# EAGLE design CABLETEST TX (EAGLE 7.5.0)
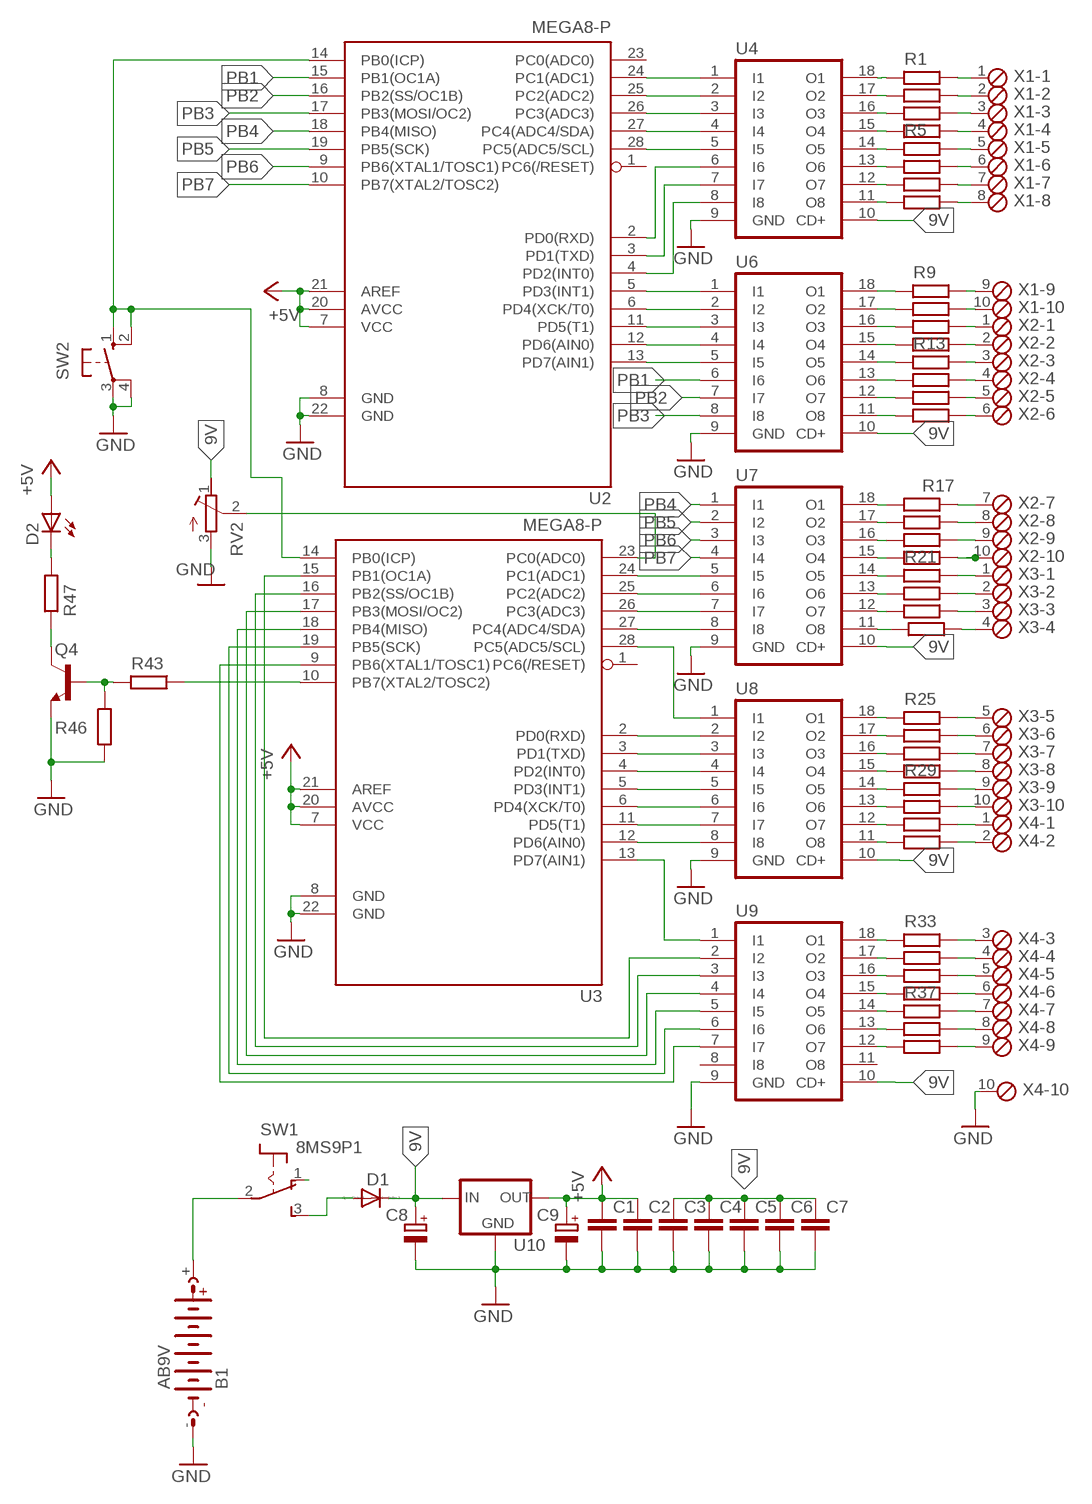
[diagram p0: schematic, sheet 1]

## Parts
B1  AB9V  [AB9V]
C1  C-EUC1206  [C1206]
C2  C-EUC1206  [C1206]
C3  C-EUC1206  [C1206]
C4  C-EUC1206  [C1206]
C5  C-EUC1206  [C1206]
C6  C-EUC1206  [C1206]
C7  C-EUC1206  [C1206]
C8  CPOL-EUE2-5  [E2-5]
C9  CPOL-EUE2-5  [E2-5]
D1  1N4004  [DO41-10]
D2  LED5MM  [LED5MM]
Q4  BC337  [TO92]
R1  R-EU_R1206  [R1206]
R2  R-EU_R1206  [R1206]
R3  R-EU_R1206  [R1206]
R4  R-EU_R1206  [R1206]
R5  R-EU_R1206  [R1206]
R6  R-EU_R1206  [R1206]
R7  R-EU_R1206  [R1206]
R8  R-EU_R1206  [R1206]
R9  R-EU_R1206  [R1206]
R10  R-EU_R1206  [R1206]
R11  R-EU_R1206  [R1206]
R12  R-EU_R1206  [R1206]
R13  R-EU_R1206  [R1206]
R14  R-EU_R1206  [R1206]
R15  R-EU_R1206  [R1206]
R16  R-EU_R1206  [R1206]
R17  R-EU_R1206  [R1206]
R18  R-EU_R1206  [R1206]
R19  R-EU_R1206  [R1206]
R20  R-EU_R1206  [R1206]
R21  R-EU_R1206  [R1206]
R22  R-EU_R1206  [R1206]
R23  R-EU_R1206  [R1206]
R24  R-EU_R1206  [R1206]
R25  R-EU_R1206  [R1206]
R26  R-EU_R1206  [R1206]
R27  R-EU_R1206  [R1206]
R28  R-EU_R1206  [R1206]
R29  R-EU_R1206  [R1206]
R30  R-EU_R1206  [R1206]
R31  R-EU_R1206  [R1206]
R32  R-EU_R1206  [R1206]
R33  R-EU_R1206  [R1206]
R34  R-EU_R1206  [R1206]
R35  R-EU_R1206  [R1206]
R36  R-EU_R1206  [R1206]
R37  R-EU_R1206  [R1206]
R38  R-EU_R1206  [R1206]
R39  R-EU_R1206  [R1206]
R43  R-EU_R1206  [R1206]
R46  R-EU_R1206  [R1206]
R47  R-EU_R1206  [R1206]
RV2  R-TRIMM-3386-F  [R-TRIMM-3386F]
SW1  8MS9P1  [8MS9]
SW2  10-XX  [B3F-10XX]
U2  MEGA8-P  [DIL28-3]
U3  MEGA8-P  [DIL28-3]
U4  ULN2803A  [DIL18]
U6  ULN2803A  [DIL18]
U7  ULN2803A  [DIL18]
U8  ULN2803A  [DIL18]
U9  ULN2803A  [DIL18]
U10  78XXL  [78XXL]
X1  MPT10  [10POL254]
X2  MPT10  [10POL254]
X3  MPT10  [10POL254]
X4  MPT10  [10POL254]

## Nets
9V: C3.1 C4.1 C5.1 C6.1 C7.1 C8.+ D1.C RV2.1(A) U4.10(CD+) U6.10(CD+) U7.10(CD+) U8.10(CD+) U9.10(CD+) U10.IN
+5V: C1.1 C2.1 C9.+ D2.A U2.7(VCC) U2.20(AVCC) U2.21(AREF) U3.7(VCC) U3.20(AVCC) U3.21(AREF) U10.OUT
GND: B1.- C1.2 C2.2 C3.2 C4.2 C5.2 C6.2 C7.2 C8.- C9.- Q4.1(E) R46.2 RV2.3(E) SW2.3(P) SW2.4(P1) U2.8(GND) U2.22(GND) U3.8(GND) U3.22(GND) U4.9(GND) U6.9(GND) U7.9(GND) U8.9(GND) U9.9(GND) U10.GND X4.10
N$1: U2.24(PC1(ADC1)) U4.1(I1)
N$2: U2.25(PC2(ADC2)) U4.2(I2)
N$3: U2.26(PC3(ADC3)) U4.3(I3)
N$4: U2.27(PC4(ADC4/SDA)) U4.4(I4)
N$5: U2.28(PC5(ADC5/SCL)) U4.5(I5)
N$6: U2.2(PD0(RXD)) U4.6(I6)
N$7: U2.3(PD1(TXD)) U4.7(I7)
N$8: U2.4(PD2(INT0)) U4.8(I8)
N$9: U2.5(PD3(INT1)) U6.1(I1)
N$10: U2.6(PD4(XCK/T0)) U6.2(I2)
N$11: U2.11(PD5(T1)) U6.3(I3)
N$12: U2.12(PD6(AIN0)) U6.4(I4)
N$13: U2.13(PD7(AIN1)) U6.5(I5)
N$14: U3.24(PC1(ADC1)) U7.5(I5)
N$15: U3.25(PC2(ADC2)) U7.6(I6)
N$16: U3.26(PC3(ADC3)) U7.7(I7)
N$17: U3.27(PC4(ADC4/SDA)) U7.8(I8)
N$18: U3.28(PC5(ADC5/SCL)) U8.1(I1)
N$19: U3.2(PD0(RXD)) U8.2(I2)
N$20: U3.3(PD1(TXD)) U8.3(I3)
N$21: U3.4(PD2(INT0)) U8.4(I4)
N$22: U3.5(PD3(INT1)) U8.5(I5)
N$23: U3.6(PD4(XCK/T0)) U8.6(I6)
N$24: U3.11(PD5(T1)) U8.7(I7)
N$25: U3.12(PD6(AIN0)) U8.8(I8)
N$26: U3.13(PD7(AIN1)) U9.1(I1)
N$27: U3.15(PB1(OC1A)) U9.2(I2)
N$28: U3.16(PB2(SS/OC1B)) U9.3(I3)
N$29: U3.17(PB3(MOSI/OC2)) U9.4(I4)
N$30: U3.18(PB4(MISO)) U9.5(I5)
N$31: U3.19(PB5(SCK)) U9.6(I6)
N$32: U3.9(PB6(XTAL1/TOSC1)) U9.7(I7)
N$33: Q4.3(C) R47.2
N$34: D1.A SW1.3(S)
N$35: RV2.2(S) U3.23(PC0(ADC0))
N$36: D2.K(C) R47.1
N$38: Q4.2(B) R43.2 R46.1
N$39: R43.1 U3.10(PB7(XTAL2/TOSC2))
N$40: SW2.1(S) SW2.2(S1) U2.14(PB0(ICP)) U3.14(PB0(ICP))
N$41: R1.2 U4.18(O1)
N$42: R1.1 X1.1
N$43: R2.2 U4.17(O2)
N$44: R2.1 X1.2
N$45: R3.2 U4.16(O3)
N$46: R3.1 X1.3
N$47: R4.1 X1.4
N$48: R5.1 X1.5
N$49: R6.1 X1.6
N$50: R8.2 U4.11(O8)
N$51: R4.2 U4.15(O4)
N$52: R5.2 U4.14(O5)
N$53: R6.2 U4.13(O6)
N$54: R7.2 U4.12(O7)
N$55: R7.1 X1.7
N$56: R8.1 X1.8
N$57: R9.1 X1.9
N$58: R10.1 X1.10
N$59: R11.1 X2.1
N$60: R12.1 X2.2
N$61: R13.1 X2.3
N$62: R14.1 X2.4
N$63: R15.1 X2.5
N$64: R16.1 X2.6
N$65: R17.2 U7.18(O1)
N$66: R18.2 U7.17(O2)
N$67: R19.2 U7.16(O3)
N$68: R20.2 U7.15(O4)
N$69: R21.2 U7.14(O5)
N$70: R22.2 U7.13(O6)
N$71: R23.2 U7.12(O7)
N$72: R24.2 U7.11(O8)
N$73: R9.2 U6.18(O1)
N$74: R10.2 U6.17(O2)
N$75: R11.2 U6.16(O3)
N$76: R12.2 U6.15(O4)
N$77: R13.2 U6.14(O5)
N$78: R14.2 U6.13(O6)
N$79: R15.2 U6.12(O7)
N$80: R16.2 U6.11(O8)
N$81: R25.1 X3.5
N$82: R17.1 X2.7
N$83: R26.1 X3.6
N$84: R18.1 X2.8
N$85: R27.1 X3.7
N$86: R19.1 X2.9
N$87: R20.1 X2.10
N$88: R21.1 X3.1
N$89: R22.1 X3.2
N$90: R28.1 X3.8
N$91: R29.1 X3.9
N$92: R30.1 X3.10
N$93: R31.1 X4.1
N$94: R32.1 X4.2
N$95: R23.1 X3.3
N$96: R24.1 X3.4
N$97: SW1.1(O)
N$98: R25.2 U8.18(O1)
N$99: R33.1 X4.3
N$100: R26.2 U8.17(O2)
N$101: R34.1 X4.4
N$102: R27.2 U8.16(O3)
N$103: R35.1 X4.5
N$104: R36.1 X4.6
N$105: R37.1 X4.7
N$106: R38.1 X4.8
N$107: R28.2 U8.15(O4)
N$108: R29.2 U8.14(O5)
N$109: R30.2 U8.13(O6)
N$110: R31.2 U8.12(O7)
N$111: R32.2 U8.11(O8)
N$112: R39.1 X4.9
N$113: B1.+ SW1.2(P)
N$114: R33.2 U9.18(O1)
N$123: R34.2 U9.17(O2)
N$124: R35.2 U9.16(O3)
N$125: R36.2 U9.15(O4)
N$126: R37.2 U9.14(O5)
N$127: R38.2 U9.13(O6)
N$128: R39.2 U9.12(O7)
PB1: U2.15(PB1(OC1A)) U6.6(I6)
PB2: U2.16(PB2(SS/OC1B)) U6.7(I7)
PB3: U2.17(PB3(MOSI/OC2)) U6.8(I8)
PB4: U2.18(PB4(MISO)) U7.1(I1)
PB5: U2.19(PB5(SCK)) U7.2(I2)
PB6: U2.9(PB6(XTAL1/TOSC1)) U7.3(I3)
PB7: U2.10(PB7(XTAL2/TOSC2)) U7.4(I4)
Unconnected: U2.1(PC6(/RESET)) U2.23(PC0(ADC0)) U3.1(PC6(/RESET)) U9.8(I8) U9.11(O8)

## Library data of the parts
B1 = battery:AB9V: 9-V BATTERY CLIP
C1-C7 = rcl:C-EU: CAPACITOR, European symbol
C8 C9 = rcl:CPOL-EU: POLARIZED CAPACITOR, European symbol
D1 = diode:1N4004: DIODE
D2 = led:LED: LED
Q4 = transistor:BC337: NPN TRANSISTOR
R1-R39 R43 R46 R47 = rcl:R-EU_: RESISTOR, European symbol
RV2 = rcl:R-TRIMM-3386-F
SW1 = switch:8MS9P1
SW2 = switch-omron:10-XX: OMRON SWITCH; MPN: B3F-1000; OC_FARNELL: 176432; OC_NEWARK: 36M3542
U2 U3 = atmel:MEGA8-P: MICROCONTROLLER 8 Kbytes FLASH, 1 kbytes SRAM, 512 bytes EEPROM, USART, 4-channel 10 bit ADC, 2-channel 8 bit ADC Pin compatible with Atmega48, ATMega88, ATMega168 Source: avr.lbr; OC_FARNELL: unknown; OC_NEWARK: unknown
U4 U6-U9 = uln-udn:ULN2803A: DRIVER ARRAY
U10 = v-reg:78XXL: VOLTAGE REGULATOR
X1-X4 = con-phoenix-254:MPT10: PHOENIX CONNECTOR; OC_FARNELL: unknown; OC_NEWARK: unknown

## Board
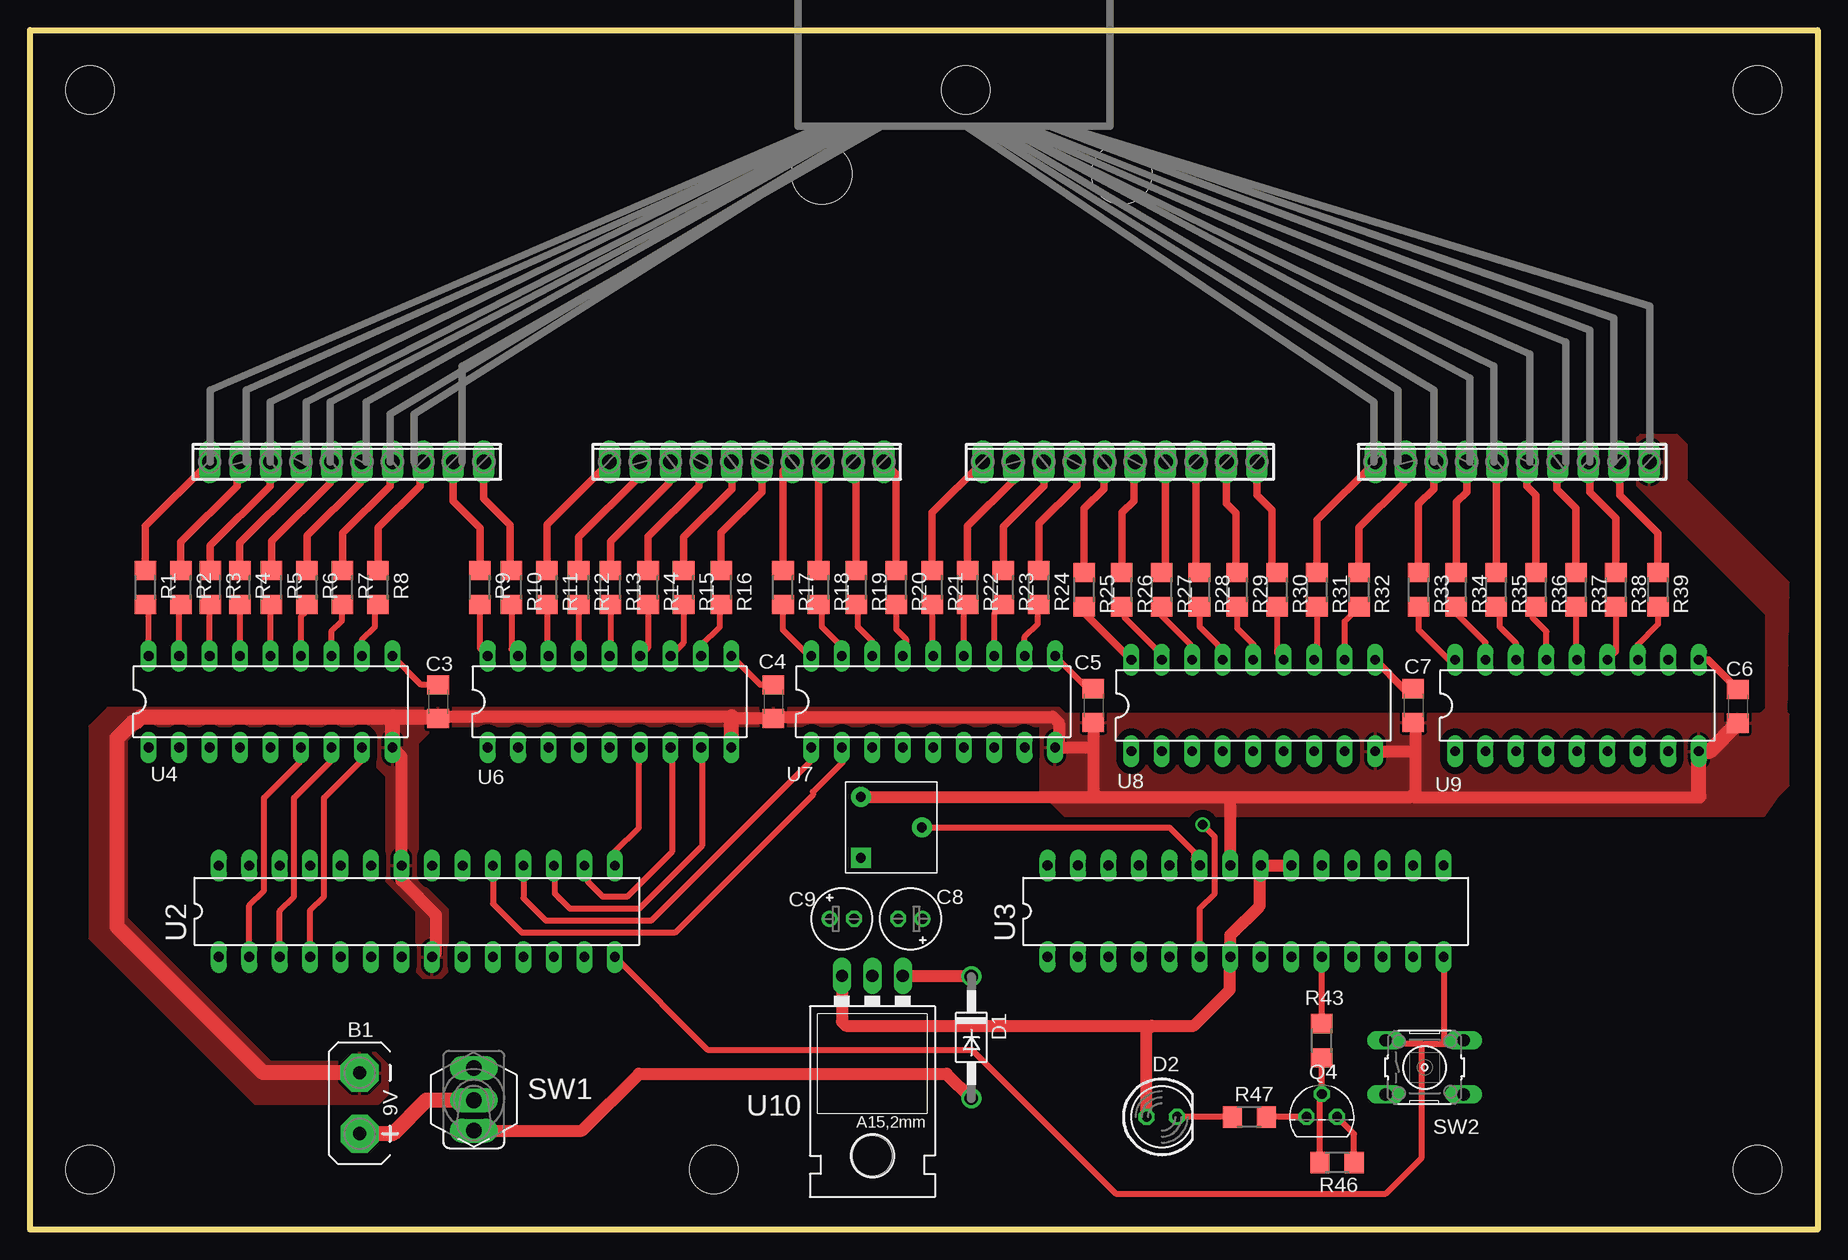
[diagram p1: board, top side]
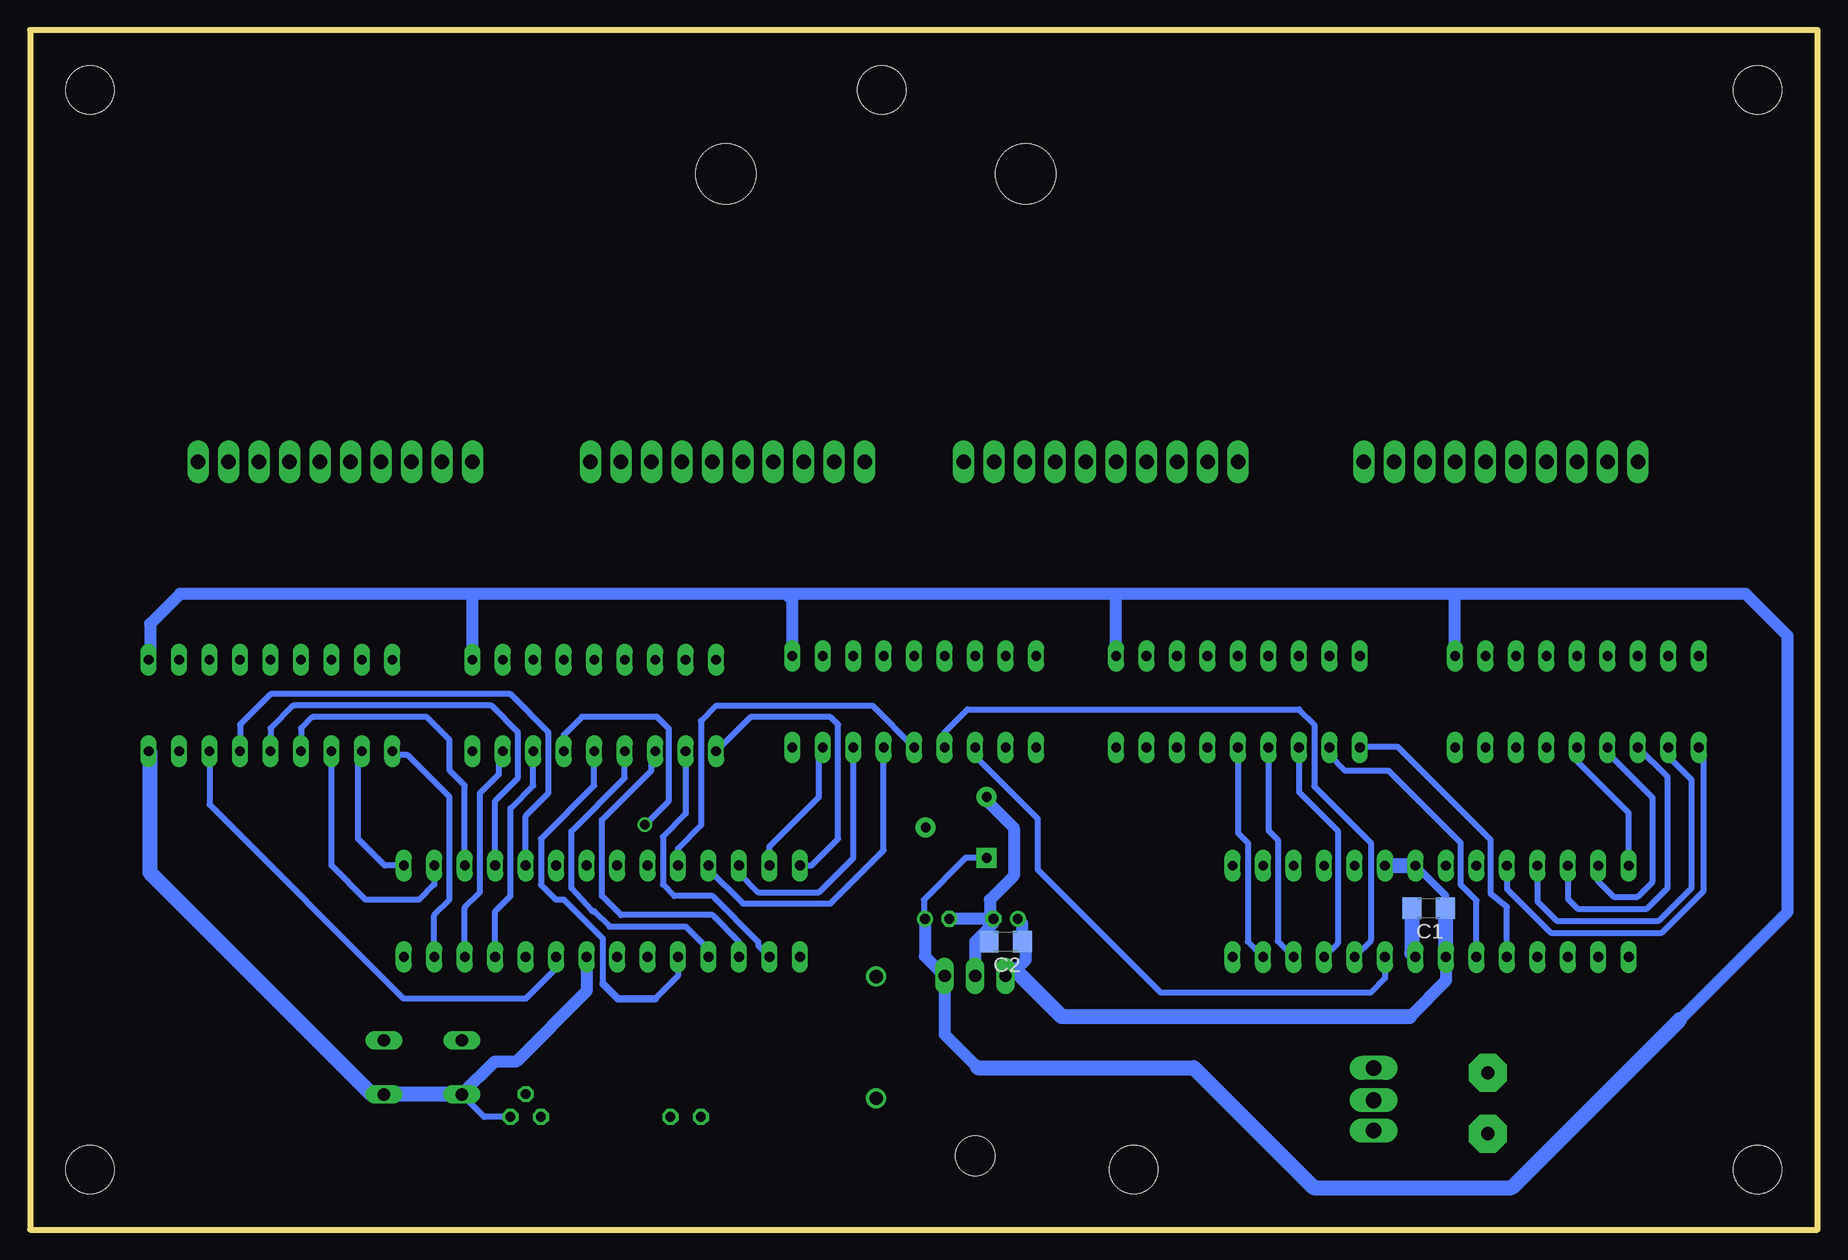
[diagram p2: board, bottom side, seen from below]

Size 149 x 100 mm. Coordinates in mm from the lower left corner, seen from the top.
Outline: 0,0 0,100 149,100 149,0 0,0
Copper layers (1*16): Top 0.035mm / dielectric 1.5mm / Bottom 0.035mm
Design rules "default": minimum track width 10mil, minimum drill 24mil, track to track 8mil, track to pad 8mil, pad to pad 8mil, via to via 8mil, smd to smd 8mil, copper to edge 40mil, drill to drill 8mil, minimum pad ring 10mil, minimum via ring 8mil, stop-mask expansion 4mil, vias tented up to drill 0mil, thermal gap 10mil
Holes 4 mm at 5,5 57,5 144,5 5,95 78,95 144,95
Holes 5 mm at 66,88 91,88

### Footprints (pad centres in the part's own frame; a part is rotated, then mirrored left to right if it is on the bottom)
AB9V = drill 1.118 pad 3.15 octagon: + 0,2.54; - 0,-2.54
C1206 = smd 1.6 x 1.8: 1 -1.4,0; 2 1.4,0
E2-5 = drill 0.813 pad 1.27: + -1.016,0 | drill 0.813 pad 1.27 octagon: - 1.016,0
DO41-10 = drill 1.118: A 5.08,0; C -5.08,0
LED5MM = drill 0.813 octagon: A -1.27,0; K 1.27,0
TO92 = drill 0.813 octagon: 1 1.27,0; 2 0,1.905; 3 -1.27,0
R1206 = smd 1.6 x 1.803: 1 -1.422,0; 2 1.422,0
R-TRIMM-3386F = drill 0.8 pad 1.676 square: 1 0,0 | drill 0.8 pad 1.676: 2 5.08,2.54; 3 0,5.08
8MS9 = drill 1.295 pad 2 long: 1 -3,5.346 | drill 1.3 pad 2 long: 2 -3,2.654; 3 -3,0.114
B3F-10XX = drill 1.016 long: 1 -3.251,2.261; 2 3.251,2.261; 3 -3.251,-2.261; 4 3.251,-2.261
DIL28-3 = drill 0.813 long: 1 -16.51,-3.81; 2 -13.97,-3.81; 3 -11.43,-3.81; 4 -8.89,-3.81; 5 -6.35,-3.81; 6 -3.81,-3.81; 7 -1.27,-3.81; 8 1.27,-3.81; 9 3.81,-3.81; 10 6.35,-3.81; 11 8.89,-3.81; 12 11.43,-3.81; 13 13.97,-3.81; 14 16.51,-3.81; 15 16.51,3.81; 16 13.97,3.81; 17 11.43,3.81; 18 8.89,3.81; 19 6.35,3.81; 20 3.81,3.81; 21 1.27,3.81; 22 -1.27,3.81; 23 -3.81,3.81; 24 -6.35,3.81; 25 -8.89,3.81; 26 -11.43,3.81; 27 -13.97,3.81; 28 -16.51,3.81
DIL18 = drill 0.813 long: 1 -10.16,-3.81; 2 -7.62,-3.81; 3 -5.08,-3.81; 4 -2.54,-3.81; 5 0,-3.81; 6 2.54,-3.81; 7 5.08,-3.81; 8 7.62,-3.81; 9 10.16,-3.81; 10 10.16,3.81; 11 7.62,3.81; 12 5.08,3.81; 13 2.54,3.81; 14 0,3.81; 15 -2.54,3.81; 16 -5.08,3.81; 17 -7.62,3.81; 18 -10.16,3.81
78XXL = drill 1.016 long: GND 0,-3.81; IN -2.54,-3.81; OUT 2.54,-3.81 | hole 3.302: 0,11.176
10POL254 = drill 1.2 long: 1 -11.43,0; 2 -8.89,0; 3 -6.35,0; 4 -3.81,0; 5 -1.27,0; 6 1.27,0; 7 3.81,0; 8 6.35,0; 9 8.89,0; 10 11.43,0

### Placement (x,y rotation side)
B1  27.48,10.53 180 top
C1  32.42,26.79 180 bottom
C2  67.67,24 180 bottom
C3  34.02,44 270 top
C4  61.96,44 270 top
C5  88.63,43.68 270 top
C6  142.35,43.61 270 top
C7  115.3,43.68 270 top
C8  73.39,25.9 180 top
C9  67.67,25.9 0 top
D1  78.47,16.02 270 top
D2  94.34,9.39 0 top
Q4  107.68,9.39 0 top
R1  9.61,53.52 270 top
R2  12.57,53.52 270 top
R3  15.03,53.52 270 top
R4  17.49,53.52 270 top
R5  20.13,53.52 270 top
R6  23.09,53.52 270 top
R7  26.05,53.52 270 top
R8  29.01,53.52 270 top
R9  37.49,53.52 270 top
R10  40.13,53.52 270 top
R11  43.09,53.52 270 top
R12  45.73,53.52 270 top
R13  48.38,53.52 270 top
R14  51.52,53.52 270 top
R15  54.48,53.52 270 top
R16  57.62,53.52 270 top
R17  62.77,53.52 270 top
R18  65.73,53.52 270 top
R19  68.87,53.52 270 top
R20  72.2,53.52 270 top
R21  75.2,53.52 270 top
R22  78.17,53.52 270 top
R23  81.12,53.52 270 top
R24  84.08,53.52 270 top
R25  87.87,53.34 270 top
R26  91.01,53.34 270 top
R27  94.34,53.34 270 top
R28  97.48,53.34 270 top
R29  100.62,53.34 270 top
R30  103.95,53.34 270 top
R31  107.27,53.34 270 top
R32  110.78,53.34 270 top
R33  115.75,53.34 270 top
R34  118.89,53.34 270 top
R35  122.22,53.34 270 top
R36  125.54,53.34 270 top
R37  128.87,53.34 270 top
R38  132.19,53.34 270 top
R39  135.7,53.34 270 top
R43  107.68,15.74 270 top
R46  108.95,5.58 0 top
R47  101.65,9.39 0 top
RV2  69.26,30.98 0 top
SW1  40,8.12 0 top
SW2  116.25,13.52 0 top
U2  32.24,26.53 0 top
U3  101.33,26.54 0 top
U4  20.05,44 0 top
U6  48.31,44 0 top
U7  75.3,44 0 top
U8  101.97,43.68 0 top
U9  128.95,43.68 0 top
U10  70.22,17.33 180 top
X1  26.4,64 0 top
X2  59.74,64 0 top
X3  90.85,64 0 top
X4  123.56,64 0 top

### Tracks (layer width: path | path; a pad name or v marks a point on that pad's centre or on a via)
9V
  Top 0.5: C3.1 32.62,45.4 U4.10 | C4.1 60.88,45.4 U6.10 | C5.1 88.18,45.08 U7.10
  Top 0.61: C7.1 114.53,45.08 U8.10 | U9.10 139.88,47.49 C6.1
  Top 1.016: U10.IN 78.43,21.14 D1.C
  Bottom 0.5: RV2.1 71.02,30.98 74.5,27.5 74.5,25.99 C8.+
  Bottom 1.016: 70,13.5 72.75,16.25 U10.IN 74.41,22.79 C8.+ | 11.5,17.5 2.5,26.5 2.5,49.5 6,53 30,53 | 30,53 58.5,53 | 58.5,53 86,53 | 86,53 112,53 | 112,53 136.5,53 139,50.5 139,47.6 U9.10 | U4.10 30.21,52.79 30,53 | U6.10 58.47,52.97 58.5,53 | U7.10 85.45,52.45 86,53 | U8.10 112.12,52.88 112,53
  Bottom 1.27: 70,13.5 52,13.5 42,3.5 25.5,3.5 11.5,17.5
+5V
  Top 1.016: 93.5,17 68,17 67.67,17.32 U10.OUT | 93.5,17 97,17 100,20 100,22.66 U3.7 100.06,24.56 102.5,27 102.5,30.25 U3.21 U3.20 | D2.A 93.08,16.57 93.5,17
  Bottom 0.61: C1.1 31.02,27.86 U2.21
  Bottom 1.016: C9.+ 66.28,25.52 C2.1 66,23.72 66,22.5 66.88,21.62 67.36,21.14 U10.OUT | U2.7 30.97,20.78 34,17.75
  Bottom 1.27: 34,17.75 63,17.75 66.88,21.62 | U2.20 U2.21 | U2.7 30.97,26.73 C1.1
GND
  Top 0.5: R46.2 110.37,7.97 Q4.1
  Top 0.61: U2.22 30.97,29.1 | 33.83,23.04 U2.8
  Top 1.016: RV2.3 89,36.06 | 89,36.06 100,36.06 | 100,36.06 115.06,36.06 115.25,36.25 | 115.25,36.25 115.5,36.5 115.5,40 | 115.5,40 115.5,42.08 C7.2 | 139.11,36.11 139,36 115.5,36 115.25,36.25 | U3.22 100.06,36 100,36.06 | C5.2 88.63,40.5 | 88.63,40.5 88.63,36.43 89,36.06 | U7.9 86,40.19 | 86,40.19 88.32,40.19 88.63,40.5 | U8.9 115.37,39.87 115.5,40 | 58.5,42.75 34.17,42.75 C3.2 | 86,40.19 85.75,40.44 85.75,42.25 85.25,42.75 62,42.75 61.96,42.71 C4.2 58.56,42.6 58.47,42.5 | U2.22 30.97,39.42 U4.9 | 30.97,29.1 33.83,26.25 33.83,23.04
  Top 1.27: 139.11,36.11 U9.9 140.01,39.87 C6.2 | U6.9 58.47,42.5 58.47,42.72 58.5,42.75 | B1.- 19.43,13.06 7.25,25.25 7.25,41 8.5,42.25 8.75,42.25 9.25,42.75 30.25,42.75 | 30.25,42.75 33.87,42.75 C3.2 | U4.9 30.21,42.71 30.25,42.75
  Bottom 0.5: Q4.1 111.13,9.39 SW2.3
  Bottom 1.016: C9.- C8.- | C2.2 69.08,25.52 C9.- | C9.- 68.69,25.52 70.22,24 U10.GND | RV2.3 69.26,35.76 67,33.5 67,29.5 69,27.5 69,26.21 C9.- | U3.8 102.6,19.9 108.5,14 110.26,14 SW2.3
  Bottom 1.27: U9.9 139,39.76 139,29.75 120.51,11.26 SW2.4 SW2.3 | C1.2 33.83,23.04 U2.8
  pour Top (isolate 0.61): 140.25,37.75 140.5,37.5 140.5,34.75 140.25,34.5
  pour Top (isolate 0.61): 138.25,41.75 139.5,43 144.25,43 144.75,43.5 144.75,51.25 134,62 134,66 134.25,66.25 137.25,66.25 138,65.5 138,62.5 146.5,54 146.25,37 144.5,34.5 138.25,34.5
  pour Top (isolate 0.61): 138.75,34.5 86.25,34.5 84.25,36.5 84.25,42 33.75,42 32.25,40.5 32.25,29.25 34.75,26.75 34.75,21.5 34.25,21 33,21 32.75,21 32.25,21.5 32.25,26.5 30.25,28.5 29.75,29 29.75,37.75 29,38.5 29,41 28,42 9.25,42 8,40.75 8,26 20,14 26.25,14 27,14.75 28.75,14.75 29.75,13.75 29.75,11.25 29.5,11 29,10.5 18.75,10.5 5,24.25 5,42 6.5,43.5 85.75,43.5 86.25,43 146.5,43 146.5,37 145.5,36 144,34.5
N$1
  Bottom 0.5: U2.24 25.89,28.39 22.25,24.75 13,24.75 9.5,28.25 9.5,39.8 U4.1
N$2
  Bottom 0.5: U2.25 23.35,27.35 21.75,25.75 13.25,25.75 10.5,28.5 10.5,37.5 12.5,39.5 12.5,40.12 U4.2
N$3
  Bottom 0.5: U4.3 12.5,37.72 12.5,28.5 14.25,26.75 20,26.75 20.81,27.56 U2.26
N$4
  Bottom 0.5: U2.27 18.27,29.02 17,27.75 15,27.75 13.75,29 13.75,36 17.25,39.5 17.25,39.93 U4.4
N$5
  Bottom 0.5: U2.28 15.73,34.73 20,39 20,40.14 U4.5
N$6
  Top 0.5: U2.2 18.27,27.02 19.5,28.25 19.5,36 22.5,39 22.5,40.1 U4.6
N$7
  Top 0.5: U2.3 20.81,26.56 22,27.75 22,36 25,39 25,40.06 U4.7
N$8
  Top 0.5: U2.4 23.35,26.6 24.5,27.75 24.5,36 27.75,39.25 27.75,40.11 U4.8
N$9
  Bottom 0.5: U2.5 25.89,26.89 27.25,28 27.25,32.5 35,40.25 38.09,40.25 U6.1
N$10
  Bottom 0.5: U6.2 40.69,39.55 39.38,38.25 35.75,38.25 29.75,32.25 29.75,28.75 28.43,27.43 U2.6
N$11
  Bottom 0.5: U6.3 43.23,36.48 40,33.25 40,23.86 U2.11
N$12
  Bottom 0.5: U6.4 45.77,33.27 45,32.5 45,24.05 U2.12
N$13
  Bottom 0.5: U6.5 48.31,33.06 47.5,32.25 47.5,24.01 U2.13
N$14
  Bottom 0.5: U7.5 78.79,43.68 91.81,43.68 93.08,42.41 93.08,33.67 95,31.75 95,30.36 U3.24
N$15
  Bottom 0.5: U3.25 92.44,30.03 89.58,27.17 82.28,27.17 77.83,31.61 U7.6
N$16
  Bottom 0.5: U3.26 89.9,29.71 88.31,28.12 83.23,28.12 80.38,30.98 U7.7
N$17
  Bottom 0.5: U3.27 87.36,31.93 83.23,36.06 83.23,39.87 U7.8
N$18
  Bottom 0.5: U8.1 88.95,42.73 82.28,42.73 81.64,42.09 81.64,32.57 83.87,30.34 U3.28
N$19
  Bottom 0.5: U3.2 88.31,23.68 88.31,24 92.12,27.8 95.3,27.8 96.25,28.76 96.25,32.75 94.34,34.66 U8.2
N$20
  Bottom 0.5: U3.3 89.9,24 92.12,26.22 99.74,26.22 101.33,27.8 101.33,34.16 97.2,38.28 97.2,39.55 U8.3
N$21
  Bottom 0.5: U3.4 92.44,23.36 94.34,25.27 100.69,25.27 101.97,26.54 102.13,26.54 102.2,26.61 103.87,28.44 103.87,33.2 99.42,37.65 U8.4
N$22
  Bottom 0.5: U3.5 94.98,21.14 96.89,19.23 | U8.5 101.97,37.01 106.41,32.57 106.41,28.75 105.16,27.5 104.5,27.5 101.25,24.25 101.25,20.5
  Bottom 0.61: 96.89,19.23 99.98,19.23 101.25,20.5
N$23  (via drill 0.8)
  Top 0.5: U3.6 97.52,26.77 98.75,28 98.75,32.75 v97.75,33.75
  Bottom 0.5: U8.6 104.5,41.25 103,42.75 96.75,42.75 95.75,41.75 95.75,35.75 v97.75,33.75
N$24
  Bottom 0.5: U3.11 110.22,26.54 108.95,27.8 108.95,35.11 107.05,37.01 U8.7
N$25
  Bottom 0.5: U3.12 112.76,26.85 111.49,28.12 111.49,36.38 109.9,37.97 109.9,39.55 U8.8
N$26
  Bottom 0.5: U3.13 115.3,26.22 114.03,27.49 114.03,36.06 117.52,39.55 118.47,39.55 U9.1
N$27
  Bottom 0.5: U3.15 119.43,30.34 121.65,32.57 121.65,39.55 U9.2
N$28
  Bottom 0.5: U3.16 115.3,28.76 116.57,27.49 121.02,27.49 123.87,30.34 U9.3
N$29
  Bottom 0.5: U3.17 112.76,37.01 114.03,38.28 114.03,40.82 115.94,42.73 125.46,42.73 126.41,41.77 U9.4
N$30
  Bottom 0.5: U3.18 110.22,35.74 108.31,37.65 108.31,41.46 110.54,43.68 127.05,43.68 128.95,41.77 U9.5
N$31
  Bottom 0.5: U3.19 107.68,34.47 105.78,36.38 105.78,41.46 108.95,44.63 128.95,44.63 131.49,42.09 U9.6
N$32
  Bottom 0.5: U3.9 105.14,21.77 107.68,19.23 117.84,19.23 134.03,35.42 U9.7
N$33
  Top 0.5: Q4.3 R47.2
N$34
  Top 1.016: SW1.3 45.98,8.23 50.75,13 76.41,13 D1.A 78.41,11
N$35
  Top 0.5: RV2.2 94.98,33.52 97,31.5 97,30.86 U3.23
N$36
  Top 0.5: R47.1 D2.K
N$38
  Top 0.5: R46.1 107.53,11.14 Q4.2 R43.2
N$39
  Top 0.5: R43.1 U3.10
N$40
  Top 0.5: 116,15.5 116,6 113,3 90.5,3 78.5,15 56.48,15 U2.14 | 116,15.5 113.28,15.5 SW2.1 | 116,15.5 117.75,15.5 | 117.75,15.5 119.23,15.5 SW2.2 | U3.14 117.84,15.59 117.75,15.5
N$41
  Top 0.5: U4.18 9.89,51.82 R1.2
N$42
  Top 0.61: R1.1 9.61,58.64 X1.1
N$43
  Top 0.5: U4.17 12.43,51.96 R2.2
N$44
  Top 0.61: R2.1 12.57,57.32 17.25,62 17.25,63.74 X1.2
N$45
  Top 0.5: U4.16 14.97,52.04 R3.2
N$46
  Top 0.61: R3.1 15.03,57.03 20,62 20,63.95 X1.3
N$47
  Top 0.61: R4.1 17.49,57.24 22.5,62.25 22.5,63.91 X1.4
N$48
  Top 0.61: R5.1 20.13,57.38 25,62.25 25,63.87 X1.5
N$49
  Top 0.61: R6.1 23.09,57.84 27.5,62.25 27.5,63.83 X1.6
N$50
  Top 0.5: U4.11 27.67,49.17 28.75,50.25 28.75,51.84 R8.2
N$51
  Top 0.5: U4.15 17.51,52.08 R4.2
N$52
  Top 0.5: U4.14 20.05,52.02 R5.2
N$53
  Top 0.5: U4.13 22.59,51.09 23,51.5 23,52.01 R6.2
N$54
  Top 0.5: U4.12 25.13,49.88 26,50.75 26,52.05 R7.2
N$55
  Top 0.61: R7.1 26.05,58.05 30,62 30,63.79 X1.7
N$56
  Top 0.61: R8.1 29.01,58.51 32.5,62 32.5,63.75 X1.8
N$57
  Top 0.61: X1.9 35.29,60.71 37.5,58.5 37.5,54.96 R9.1
N$58
  Top 0.61: X1.10 37.83,60.92 40,58.75 40,55.08 R10.1
N$59
  Top 0.61: R11.1 43.09,58.78 X2.1
N$60
  Top 0.61: R12.1 45.73,57.73 50.75,62.75 50.75,63.9 X2.2
N$61
  Top 0.61: R13.1 48.38,57.38 53.25,62.25 53.25,63.86 X2.3
N$62
  Top 0.61: R14.1 51.52,57.77 55.75,62 55.75,63.82 X2.4
N$63
  Top 0.61: R15.1 54.48,57.73 58.5,61.75 58.5,63.97 X2.5
N$64
  Top 0.61: R16.1 57.62,58.12 61,61.5 X2.6
N$65
  Top 0.5: U7.18 64.94,47.81 62.75,50 62.75,52.08 R17.2
N$66
  Top 0.5: U7.17 67.67,48.58 66,50.25 66,51.83 R18.2
N$67
  Top 0.5: U7.16 70.22,49.03 69,50.25 69,51.97 R19.2
N$68
  Top 0.5: R20.2 72.2,50.05 73,49.25 73,48.05 U7.15
N$69
  Top 0.5: R21.2 75.2,47.9 U7.14
N$70
  Top 0.5: U7.13 77.83,51.77 R22.2
N$71
  Top 0.5: U7.12 80.38,51.35 R23.2
N$72
  Top 0.5: U7.11 82.92,49.41 84,50.5 84,52.02 R24.2
N$73
  Top 0.5: R9.2 37.49,48.47 U6.18
N$74
  Top 0.5: R10.2 40.13,48.37 U6.17
N$75
  Top 0.5: R11.2 43.09,47.95 U6.16
N$76
  Top 0.5: R12.2 45.73,47.84 U6.15
N$77
  Top 0.5: R13.2 48.38,47.88 U6.14
N$78
  Top 0.5: R14.2 51.52,48.48 U6.13
N$79
  Top 0.5: R15.2 54.48,48.9 U6.12
N$80
  Top 0.5: U6.11 55.93,48.68 57.5,50.25 57.5,51.98 R16.2
N$81
  Top 0.61: R25.1 87.87,60.12 89.5,61.75 89.5,63.92 X3.5
N$82
  Top 0.61: R17.1 62.77,63.22 X2.7
N$83
  Top 0.61: R26.1 91.01,59.76 92,60.75 92,63.88 X3.6
N$84
  Top 0.61: R18.1 65.73,63.64 X2.8
N$85
  Top 0.61: X3.7 94.66,55.09 R27.1
N$86
  Top 0.61: R19.1 68.87,63.76 X2.9
N$87
  Top 0.61: R20.1 72.2,62.97 X2.10
N$88
  Top 0.61: R21.1 75.2,59.78 X3.1
N$89
  Top 0.61: R22.1 78.17,58.66 82,62.5 82,63.96 X3.2
N$90
  Top 0.61: X3.8 97.2,55.04 R28.1
N$91
  Top 0.61: X3.9 99.74,60.51 100.5,59.75 100.5,54.88 R29.1
N$92
  Top 0.61: X3.10 102.28,61.22 103.5,60 103.5,55.21 R30.1
N$93
  Top 0.61: R31.1 107.27,59.15 X4.1
N$94
  Top 0.61: R32.1 110.78,58.53 114.5,62.25 114.5,63.84 X4.2
N$95
  Top 0.61: R23.1 81.12,58.62 84.5,62 X3.3
N$96
  Top 0.61: R24.1 84.08,58.84 87.25,62 87.25,63.79 X3.4
N$98
  Top 0.61: R25.2 87.87,51.42 U8.18
N$99
  Top 0.61: R33.1 115.75,60.5 117,61.75 117,63.8 X4.3
N$100
  Top 0.5: U8.17 94.34,47.91 91.25,51 91.25,51.68 R26.2
N$101
  Top 0.61: R34.1 118.89,60.64 119.75,61.5 X4.4
N$102
  Top 0.5: R27.2 94.34,51.16 96.75,48.75 96.75,47.62 U8.16
N$103
  Top 0.61: R35.1 122.22,63.93 X4.5
N$104
  Top 0.61: R36.1 125.54,61.21 124.75,62 124.75,63.92 X4.6
N$105
  Top 0.61: R37.1 128.87,60.13 127.25,61.75 127.25,63.88 X4.7
N$106
  Top 0.61: R38.1 132.19,59.31 130,61.5 130,63.91 X4.8
N$107
  Top 0.5: R28.2 97.48,50.27 99,48.75 99,47.91 U8.15
N$108
  Top 0.5: R29.2 100.62,50.13 102,48.75 102,47.52 U8.14
N$109
  Top 0.5: R30.2 103.95,48.05 U8.13
N$110
  Top 0.5: R31.2 107.27,47.72 U8.12
N$111
  Top 0.5: U8.11 109.58,50.72 R32.2
N$112
  Top 0.61: R39.1 135.7,58.05 132.5,61.25 132.5,63.95 X4.9
N$113
  Top 1.27: SW1.2 33.02,10.77 30.25,8 27.5,8 B1.+
N$114
  Top 0.5: U9.18 118.26,47.49 115.75,50 R33.2
N$123
  Top 0.5: U9.17 121.33,48.92 119,51.25 119,51.81 R34.2
N$124
  Top 0.5: U9.16 123.87,48.88 122.5,50.25 122.5,51.63 R35.2
N$125
  Top 0.5: U9.15 126.41,49.84 125.25,51 125.25,51.63 R36.2
N$126
  Top 0.5: R37.2 128.87,47.58 U9.14
N$127
  Top 0.5: R38.2 132.19,48.19 U9.13
N$128
  Top 0.5: R39.2 135.7,50.45 134,48.75 134,47.52 U9.12
PB1
  Top 0.5: U2.15 48.75,31.5 50.75,33.5 50.75,40.09 U6.6
PB2
  Top 0.5: U6.7 53.5,40.08 53.5,31.5 49.75,27.75 47.75,27.75 46.5,29 46.5,30.05 U2.16
PB3
  Top 0.5: 43.67,29.33 U2.17 43.75,30.27 43.75,28 45,26.75 50.75,26.75 56,32 56,40.12 U6.8
PB4
  Top 0.5: U2.18 41.13,27.62 43,25.75 51.75,25.75 65,39 65,40.05 U7.1
PB5
  Top 0.5: U2.19 38.59,27.16 41,24.75 53.75,24.75 65.25,36.25 65.25,36.5 67.75,39 67.75,40.11 U7.2
PB6
  Bottom 0.5: U2.9 36.05,20.95 37.25,19.75 54.75,19.75 65,30 65,34.25 70,39.25 70,39.97 U7.3
PB7
  Bottom 0.5: U7.4 72.75,41.46 70.85,43.36 43.23,43.36 41.96,42.09 41.96,36.96 37.25,32.25 37.25,24.07 U2.10

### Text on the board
tDocu: - - - - - - - - - - - - - - - - - - - - - - - - - - - - -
